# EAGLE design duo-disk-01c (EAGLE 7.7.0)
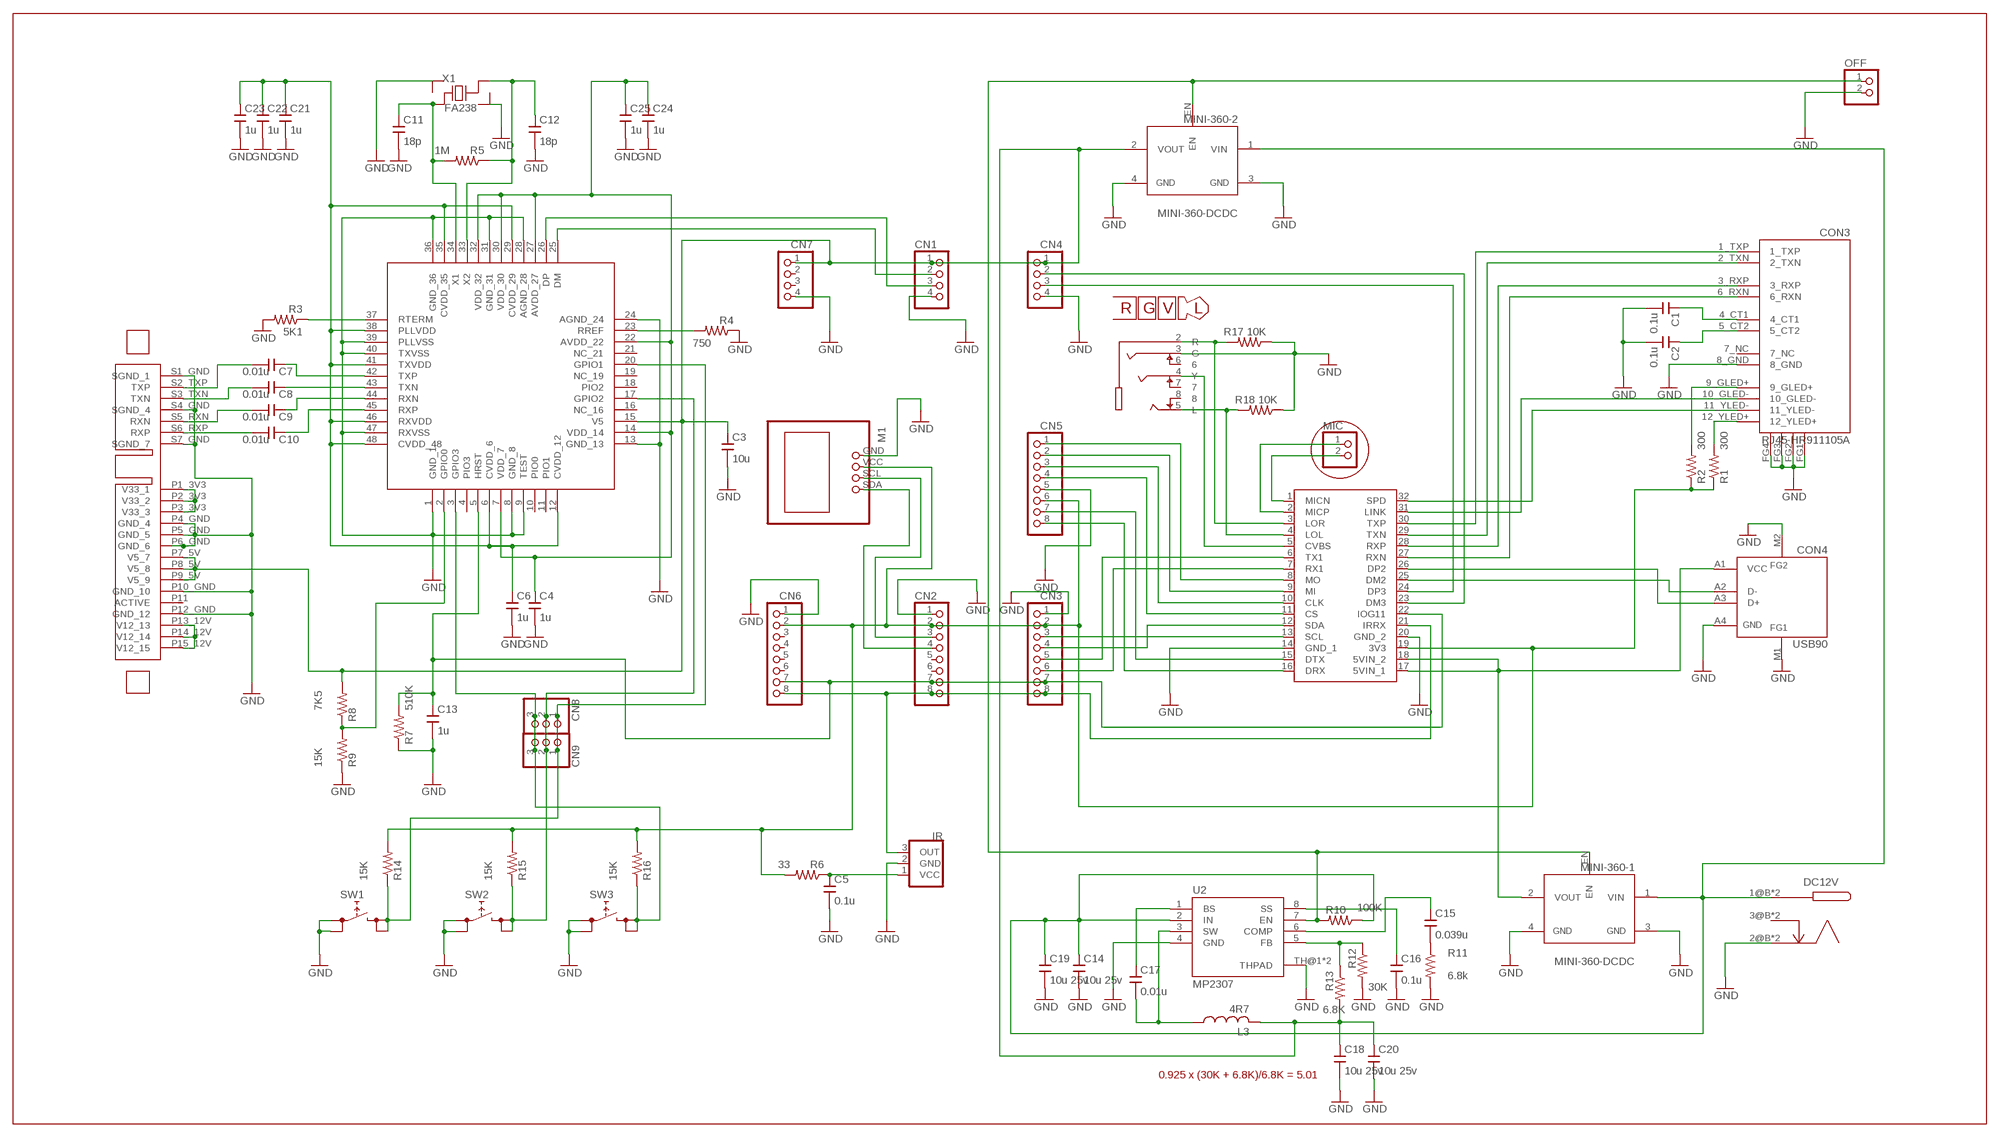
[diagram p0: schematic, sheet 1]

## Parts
C1  0.1u  C/SMDC2012  [C2012]
C2  0.1u  C/SMDC2012  [C2012]
C3  10u  C/SMDC2012  [C2012]
C4  1u  C/SMDC2012  [C2012]
C5  0.1u  C/SMDC2012  [C2012]
C6  1u  C/SMDC2012  [C2012]
C7  0.01u  C/SMDC2012  [C2012]
C8  0.01u  C/SMDC2012  [C2012]
C9  0.01u  C/SMDC2012  [C2012]
C10  0.01u  C/SMDC2012  [C2012]
C11  18p  C/SMDC2012  [C2012]
C12  18p  C/SMDC2012  [C2012]
C13  1u  C/SMDC2012  [C2012]
C14  10u 25v  C/SMDC3216  [C3216]
C15  0.039u  C/SMDC2012  [C2012]
C16  0.1u  C/SMDC2012  [C2012]
C17  0.01u  C/SMDC2012  [C2012]
C18  10u 25v  C/SMDC3216  [C3216]
C19  10u 25v  C/SMDC3216  [C3216]
C20  10u 25v  C/SMDC3216  [C3216]
C21  1u  C/SMDC2012  [C2012]
C22  1u  C/SMDC2012  [C2012]
C23  1u  C/SMDC2012  [C2012]
C24  1u  C/SMDC2012  [C2012]
C25  1u  C/SMDC2012  [C2012]
CN1  CONN4N  [PINHDR1X4]
CN2  PINHDR8  [PINHDR1X8]
CN3  PINHDR8  [PINHDR1X8]
CN4  CONN4N  [PINHDR1X4]
CN5  PINHDR8  [PINHDR1X8]
CN6  PINHDR8  [PINHDR1X8]
CN7  CONN4N  [PINHDR1X4]
CN8  PINHDR3S  [PINHDRS3]
CN9  PINHDR3P  [PADS3]
CON1  SATA-22-07  [SATA-22PIN-A07]
CON2  PJ393  [PJ393]
CON3  RJ45-HR911105A  [RJ45-HR911105A]
CON4  USB90  [USB-AF90]
DC12V  DC-JACK7  [DC-JACK7]
IR  TL1338  [TL1338]
L3  4R7  L/SMD  [L10040]
M1  OLED12864  [OLED12864]
M2  NANOPI-DUO  [NANOPI-DUO]
MIC  PINHDR2  [PINHDR2]
MINI-360-1  MINI-360-DCDC  [MINI-360-DCDC]
MINI-360-2  MINI-360-DCDC  [MINI-360-DCDC]
OFF  PINHDR2  [PINHDR2]
R1  300  R/SMDR2012  [R2012]
R2  300  R/SMDR2012  [R2012]
R3  5K1  R/SMDR2012  [R2012]
R4  750  R/SMDR2012  [R2012]
R5  1M  R/SMDR2012  [R2012]
R6  33  R/SMDR2012  [R2012]
R7  510K  R/SMDR2012  [R2012]
R8  7K5  R/SMDR2012  [R2012]
R9  15K  R/SMDR2012  [R2012]
R10  100K  R/SMDR2012  [R2012]
R11  6.8k  R/SMDR2012  [R2012]
R12  30K  R/SMDR2012  [R2012]
R13  6.8K  R/SMDR2012  [R2012]
R14  15K  R/SMDR2012  [R2012]
R15  15K  R/SMDR2012  [R2012]
R16  15K  R/SMDR2012  [R2012]
R17  10K  R/SMDR2012  [R2012]
R18  10K  R/SMDR2012  [R2012]
SW1  TACTSWSMD+  [TACTSW/SMD+]
SW2  TACTSWSMD+  [TACTSW/SMD+]
SW3  TACTSWSMD+  [TACTSW/SMD+]
U1  GL830  [TQFP48]
U2  MP2307  [SOP8PAD]
X1  FA238  [FA238]

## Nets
CLK: CN5.3 M2.10(CLK)
CS: CN5.4 M2.11(CS)
DM2: CON4.A2(D-) M2.25(DM2)
DM3: CN4.2 M2.23(DM3)
DP2: CON4.A3(D+) M2.26(DP2)
DP3: CN4.3 M2.24(DP3)
DRX: CN5.8 M2.16(DRX)
DTX: CN5.7 M2.15(DTX)
G11: C13.1 CN2.7 CN3.7 CN6.7 M2.22(IOG11) R7.2 U1.5(HRST)
GND: C1.2 C2.2 C3.2 C4.2 C5.2 C6.2 C11.2 C12.2 C13.2 C14.2 C16.2 C18.2 C19.2 C20.2 C21.2 C22.2 C23.2 C24.2 C25.2 CN1.4 CN2.1 CN3.1 CN4.4 CN5.5 CN6.1 CN7.4 CON1.P4_GND(GND_4) CON1.P5_GND(GND_5) CON1.P6_GND(GND_6) CON1.P10_GND(GND_10) CON1.P12_GND(GND_12) CON1.S1_GND(SGND_1) CON1.S4_GND(SGND_4) CON1.S7_GND(SGND_7) CON2.3(G) CON3.8_GND CON3.FG1(GND) CON3.FG2(GND) CON3.FG3(GND) CON3.FG4(GND) CON4.A4(GND) CON4.M1(GND) CON4.M2(GND) DC12V.2@B(GND) DC12V.2@T(GND) IR.2(GND) M1.GND M2.14(GND_1) M2.20(GND_2) MINI-360-1.3(GND) MINI-360-1.4(GND) MINI-360-2.3(GND) MINI-360-2.4(GND) OFF.2 R3.2 R4.1 R7.1 R9.1 R11.2 R12.2 R17.1 R18.1 SW1.1 SW1.2 SW2.1 SW2.2 SW3.1 SW3.2 U1.1(GND_1) U1.8(GND_8) U1.9(TEST) U1.13(GND_13) U1.24(AGND_24) U1.28(AGND_28) U1.31(GND_31) U1.36(GND_36) U1.39(PLLVSS) U1.40(TXVSS) U1.47(RXVSS) U2.4(GND) U2.TH@1(THPAD) U2.TH@2(THPAD) X1.2 X1.4
GPIO0: R8.1 R9.2 U1.2(GPIO0)
GPIO1: CN8.1 CN9.1 R14.1 SW1.3 SW1.4 U1.20(GPIO1)
GPIO2: CN8.2 CN9.2 R15.1 SW2.3 SW2.4 U1.17(GPIO2)
GPIO3: CN8.3 CN9.3 R16.1 SW3.3 SW3.4 U1.3(GPIO3)
IRRX: CN2.8 CN3.8 CN6.8 IR.3(OUT) M2.21(IRRX)
LINK: CON3.10_GLED- M2.31(LINK)
M3V3: CN2.2 CN3.2 CN5.6 CN6.2 M1.VCC M2.19(3V3) R1.1 R2.1 R6.2 R14.2 R15.2 R16.2
M5V: C3.1 C18.1 C20.1 CN1.1 CN4.1 CN7.1 CON1.P7_5V(V5_7) CON1.P8_5V(V5_8) CON1.P9_5V(V5_9) L3.2 L3.2B MINI-360-2.2(VOUT) R8.2 R13.2 U1.15(V5)
MI: CN5.2 M2.9(MI)
MO: CN5.1 M2.8(MO)
N$4: CN1.2 U1.25(DM)
N$7: CN1.3 U1.26(DP)
N$8: CON2.5(L) M2.4(LOL) R18.2
N$9: CON2.4(Y) M2.5(CVBS)
N$10: C17.2 L3.1 L3.1B U2.3(SW)
N$12: CON2.2(R) M2.3(LOR) R17.2
N$13: MINI-360-1.EN MINI-360-2.EN OFF.1 R10.2 U2.7(EN)
N$14: C16.1 U2.8(SS)
N$15: C15.2 R11.1
N$16: C15.1 U2.6(COMP)
N$17: R12.1 R13.1 U2.5(FB)
N$27: M2.2(MICP) MIC.1
N$28: M2.1(MICN) MIC.2
N$30: C7.1 U1.42(TXP)
N$33: C1.1 CON3.4_CT1
N$34: C2.1 CON3.5_CT2
N$36: CON3.9_GLED+ R2.2
N$37: CON3.12_YLED+ R1.2
N$38: CON1.P1_3V3(V33_1) CON1.P2_3V3(V33_2) CON1.P3_3V3(V33_3)
N$39: C17.1 U2.1(BS)
N$41: CON1.P13_12V(V12_13) CON1.P14_12V(V12_14) CON1.P15_12V(V12_15)
N$42: R3.1 U1.37(RTERM)
N$43: R4.2 U1.23(RREF)
N$46: C8.1 U1.43(TXN)
N$47: C7.2 CON1.S2_TXP(TXP)
N$48: C8.2 CON1.S3_TXN(TXN)
N$49: C9.2 CON1.S5_RXN(RXN)
N$50: C10.2 CON1.S6_RXP(RXP)
N$51: C9.1 U1.44(RXN)
N$52: C10.1 U1.45(RXP)
N$53: C11.1 R5.2 U1.34(X1) X1.1
N$54: C12.1 R5.1 U1.33(X2) X1.3
N$61: C5.1 IR.1(VCC) R6.1
OSCL: CN2.3 M1.SCL
OSDA: CN2.4 M1.SDA
RX1: CN3.6 M2.7(RX1)
RXN: CON3.6_RXN M2.27(RXN)
RXP: CON3.3_RXP M2.28(RXP)
S1V8: C6.1 C21.1 C22.1 C23.1 U1.6(CVDD_6) U1.12(CVDD_12) U1.29(CVDD_29) U1.35(CVDD_35) U1.38(PLLVDD) U1.41(TXVDD) U1.46(RXVDD) U1.48(CVDD_48)
S3V3: C4.1 C24.1 C25.1 U1.7(VDD_7) U1.14(VDD_14) U1.22(AVDD_22) U1.27(AVDD_27) U1.30(VDD_30) U1.32(VDD_32)
SCL: CN3.3 M2.13(SCL)
SDA: CN3.4 M2.12(SDA)
SPD: CON3.11_YLED- M2.32(SPD)
TX1: CN3.5 M2.6(TX1)
TXN: CON3.2_TXN M2.29(TXN)
TXP: CON3.1_TXP M2.30(TXP)
VIN: C14.1 C19.1 DC12V.1@B(VIN) DC12V.1@T(VIN) MINI-360-1.1(VIN) MINI-360-2.1(VIN) R10.1 U2.2(IN)
VOUT: CON4.A1(VCC) M2.17(5VIN_1) M2.18(5VIN_2) MINI-360-1.2(VOUT)
Unconnected: CN2.5 CN2.6 CN6.3 CN6.4 CN6.5 CN6.6 CN7.2 CN7.3 CON1.P11(ACTIVE) CON2.6 CON2.7 CON2.8 CON3.7_NC DC12V.3@B(SENSE) DC12V.3@T(SENSE) U1.4(PIO3) U1.10(PIO0) U1.11(PIO1) U1.16(NC_16) U1.18(PIO2) U1.19(NC_19) U1.21(NC_21)

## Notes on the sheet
- 0.925 x (30K + 6.8K)/6.8K = 5.01

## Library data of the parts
C1-C25 = SRT162-020:C/SMD
CN1 CN4 CN7 = SRT162-020:CONN4: connector 4
CN2 CN3 CN5 CN6 = SRT162-020:PINHDR8
CN8 CN9 = SRT162-020:PINHDR3
CON1 = SRT162-020:SATA-22
CON2 = SRT162-020:PJ393
CON3 = SRT162-020:RJ45-HR911105A
CON4 = SRT162-020:USB
DC12V = SRT162-020:DC-JACK
IR = SRT162-020:TL1338
L3 = SRT162-020:L/SMD: VLF4012AT
M1 = SRT162-020:OLED12864
M2 = SRT162-020:NANOPI-DUO
MIC OFF = SRT162-020:PINHDR2
MINI-360-1 MINI-360-2 = SRT162-020:MINI-360-DCDC
R1-R18 = SRT162-020:R/SMD
SW1-SW3 = SRT162-020:TACTSW: 4pin tactsw (1,2 - 3,4)
U1 = SRT162-020:GL830
U2 = SRT162-020:MP2307
X1 = SRT162-020:FA238

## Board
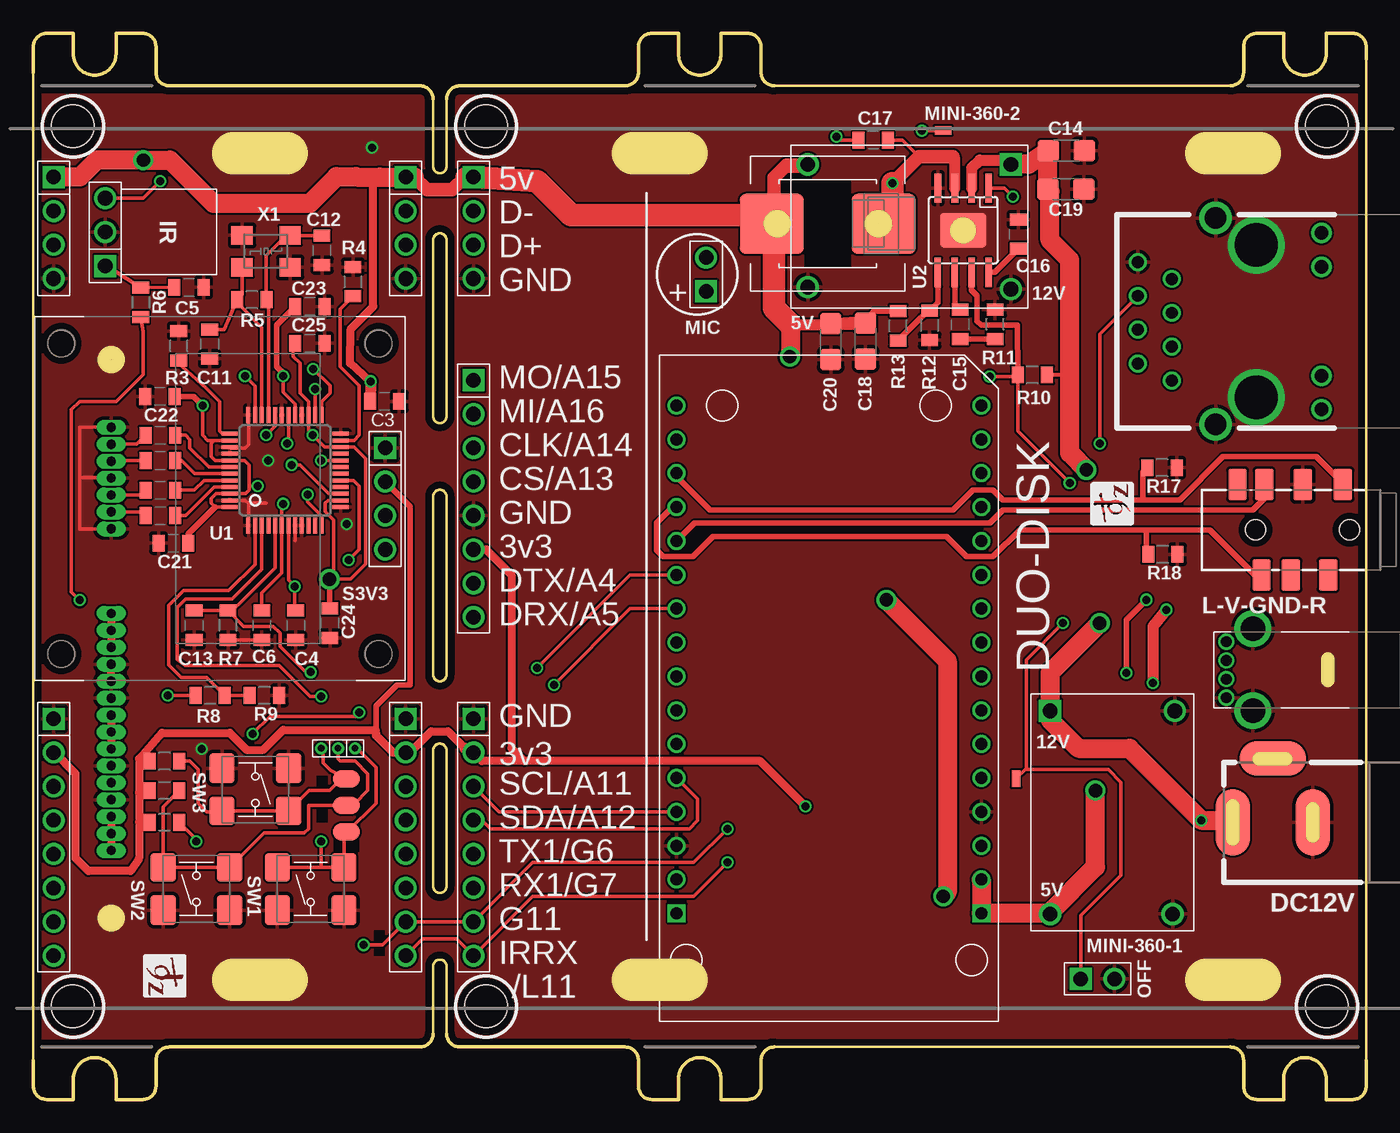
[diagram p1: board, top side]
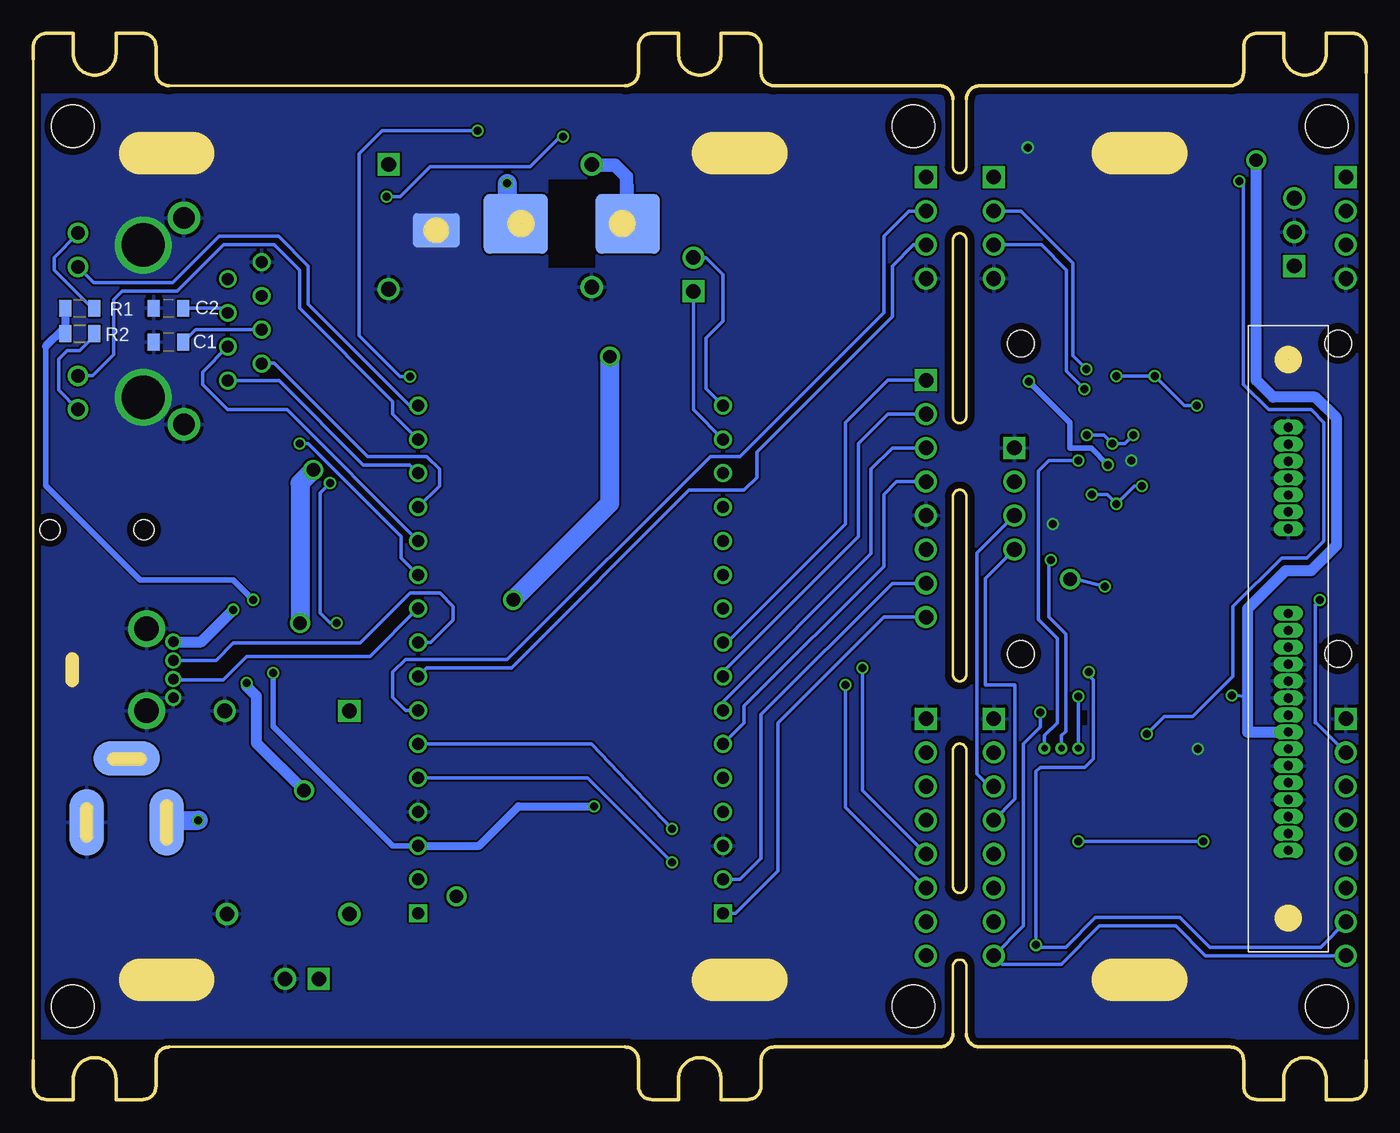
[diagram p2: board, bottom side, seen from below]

Size 100 x 80 mm. Coordinates in mm from the lower left corner, seen from the top.
Outline: 106 segments
Copper layers (1*16): Top 0.035mm / dielectric 1.6mm / Bottom 0.035mm
Design rules "Elecrow_2-layer_PCB_eagle_rule *": minimum track width 6mil, minimum drill 12mil, track to track 6mil, track to pad 6mil, pad to pad 6mil, via to via 8mil, smd to smd 0mil, copper to edge 20mil, drill to drill 10mil, minimum pad ring 8mil, minimum via ring 6mil, stop-mask expansion 0mil, vias tented up to drill 100mil, thermal gap 10mil
Holes 3.2 mm at 2.97,73.02 97.05,73.02 97.05,6.98 2.97,6.98 33.97,73.02 33.97,6.98
tRestrict: area 22.5,18.6 to 24.4,19.4; area 21.3,20.8 to 22.1,22.7; area 25.6,10.8 to 26.4,12.7; area 21.3,22.4 to 22.1,24.3; area -3,75.5 to 104,81; area -4,-1 to 103,4.5
bRestrict: area 21,28.1 to 23.8,29.2; area -3,75.5 to 104,81; area -4,-1 to 103,4.5
Milling: 6 lines

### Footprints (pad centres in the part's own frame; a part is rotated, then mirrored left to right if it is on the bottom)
C2012 = smd 0.9 x 1.25: 1 -1.1,0; 2 1.1,0
C3216 = smd 1.6 x 1.6: 1 -1.35,0; 2 1.35,0
PINHDR1X4 = drill 1.1 square: 1 -3.81,0 | drill 1.1: 2 -1.27,0; 3 1.27,0; 4 3.81,0
PINHDR1X8 = drill 1.1 square: 1 -8.89,0 | drill 1.1: 2 -6.35,0; 3 -3.81,0; 4 -1.27,0; 5 1.27,0; 6 3.81,0; 7 6.35,0; 8 8.89,0
PINHDRS3 = drill 0.5: 1 0,0; 2 1.27,0; 3 2.54,0
PADS3 = smd 1.3 x 2: 1 -2,0; 2 0,0; 3 2,0
SATA-22PIN-A07 = drill 0.7 pad 1.081 long: P1_3V3 0,0; P2_3V3 -1.27,0; P3_3V3 -2.54,0; P4_GND -3.81,0; P5_GND -5.08,0; P6_GND -6.35,0; P7_5V -7.62,0; P8_5V -8.89,0; P9_5V -10.16,0; P10_GND -11.43,0; P11 -12.7,0; P12_GND -13.97,0; P13_12V -15.24,0; P14_12V -16.51,0; P15_12V -17.78,0; S1_GND 13.97,0; S2_TXP 12.7,0; S3_TXN 11.43,0; S4_GND 10.16,0; S5_RXN 8.89,0; S6_RXP 7.62,0; S7_GND 6.35,0
PJ393 = smd 2.4 x 1.4: 2 -3.4,-2.8; 3 -3.4,-5.8; 4 -3.4,-8.7; 5 3.4,-8.9; 6 3.4,-3.9; 7 3.4,-6.7; 8 -3.4,-10.7 | hole 1.5: 0,-2.3; 0,-9.35
RJ45-HR911105A = drill 0.89: 1_TXP 4.45,-6.35; 2_TXN 3.18,-8.89; 3_RXP 1.91,-6.35; 4_CT1 0.64,-8.89; 5_CT2 -0.63,-6.35; 6_RXN -1.9,-8.89; 7_NC -3.17,-6.35; 8_GND -4.44,-8.89 | drill 1.02 pad 1.528: 9_GLED+ 6.625,4.9; 10_GLED- 4.085,4.9; 11_YLED- -4.085,4.9; 12_YLED+ -6.625,4.9 | drill 1.63: FG1 7.745,-3.05; FG2 -7.745,-3.05 | drill 3.25 pad 3.75: FG3 5.715,0; FG4 -5.715,0
USB-AF90 = drill 0.8 pad 1.156: A1 2,-2.1; A2 2,-0.7; A3 2,0.7; A4 2,2.1 | drill 1.84 pad 2.348: M1 0,3.08; M2 0,-3.08
DC-JACK7 = smd 2.6 x 5 bottom: 1@B 4,0; 2@B -2,0 | smd 2.6 x 5: 1@T 4,0; 2@T -2,0 | smd 5 x 2.6 bottom: 3@B 1,-4.8 | smd 5 x 2.6: 3@T 1,-4.8
TL1338 = drill 1.1 square: 1 2.54,0 | drill 1.1: 2 0,0; 3 -2.54,0
L10040 = smd 4.5 x 4.8: 1 0,4.2; 2 0,-4.2 | smd 4.5 x 4.8 bottom: 1B 0,4.2; 2B 0,-4.2
OLED12864 = drill 1.1 square: GND -3.81,0 | drill 1.1: SCL 1.27,0; SDA 3.81,0; VCC -1.27,0 | hole 2: -11.65,-0.5; 11.65,-0.5; -11.65,-24.3; 11.65,-24.3
NANOPI-DUO = drill 0.9: 1 -10.16,10.16; 2 -10.16,7.62; 3 -10.16,5.08; 4 -10.16,2.54; 5 -10.16,0; 6 -10.16,-2.54; 7 -10.16,-5.08; 8 -10.16,-7.62; 9 -10.16,-10.16; 10 -10.16,-12.7; 11 -10.16,-15.24; 12 -10.16,-17.78; 13 -10.16,-20.32; 14 -10.16,-22.86; 15 -10.16,-25.4; 18 12.7,-25.4; 19 12.7,-22.86; 20 12.7,-20.32; 21 12.7,-17.78; 22 12.7,-15.24; 23 12.7,-12.7; 24 12.7,-10.16; 25 12.7,-7.62; 26 12.7,-5.08; 27 12.7,-2.54; 28 12.7,0; 29 12.7,2.54; 30 12.7,5.08; 31 12.7,7.62; 32 12.7,10.16 | drill 0.9 square: 16 -10.16,-27.94; 17 12.7,-27.94
PINHDR2 = drill 1.1 square: 1 -1.27,0 | drill 1.1: 2 1.27,0
MINI-360-DCDC = drill 1.1 pad 1.676 square: 1 -7.62,-5.08 | drill 1.1 pad 1.676: 2 7.62,-5.08; 3 7.62,4.128; 4 -7.62,4.286 | smd 1.27 x 0.66: EN -2.54,-7.62
R2012 = smd 0.9 x 1.25: 1 -1.1,0; 2 1.1,0
TACTSW/SMD+ = smd 2.25 x 1.9: 1 -1.6,2.5; 2 -1.6,-2.5 | smd 2.15 x 1.9: 3 1.6,2.5; 4 1.6,-2.5
TQFP48 = smd 1.2 x 0.3: 1 -4.15,2.75; 2 -4.15,2.25; 3 -4.15,1.75; 4 -4.15,1.25; 5 -4.15,0.75; 6 -4.15,0.25; 7 -4.15,-0.25; 8 -4.15,-0.75; 9 -4.15,-1.25; 10 -4.15,-1.75; 11 -4.15,-2.25; 12 -4.15,-2.75; 25 4.15,-2.75; 26 4.15,-2.25; 27 4.15,-1.75; 28 4.15,-1.25; 29 4.15,-0.75; 30 4.15,-0.25; 31 4.15,0.25; 32 4.15,0.75; 33 4.15,1.25; 34 4.15,1.75; 35 4.15,2.25; 36 4.15,2.75 | smd 0.3 x 1.2: 13 -2.75,-4.15; 14 -2.25,-4.15; 15 -1.75,-4.15; 16 -1.25,-4.15; 17 -0.75,-4.15; 18 -0.25,-4.15; 19 0.25,-4.15; 20 0.75,-4.15; 21 1.25,-4.15; 22 1.75,-4.15; 23 2.25,-4.15; 24 2.75,-4.15; 37 2.75,4.15; 38 2.25,4.15; 39 1.75,4.15; 40 1.25,4.15; 41 0.75,4.15; 42 0.25,4.15; 43 -0.25,4.15; 44 -0.75,4.15; 45 -1.25,4.15; 46 -1.75,4.15; 47 -2.25,4.15; 48 -2.75,4.15
SOP8PAD = smd 0.5 x 2.2: 1 -1.905,-3.154; 2 -0.645,-3.154; 3 0.625,-3.154; 4 1.895,-3.154; 5 1.905,3.154; 6 0.635,3.154; 7 -0.635,3.154; 8 -1.905,3.154 | smd 3.454 x 2.565: TH@1 0,0 | smd 3.454 x 2.565 bottom: TH@2 0,0
FA238 = smd 1.6 x 1.4: 1 -1.8,-1.2; 2 1.8,-1.2; 3 1.8,1.2; 4 -1.8,1.2

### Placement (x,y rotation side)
C1  89.85,56.83 180 bottom
C2  89.85,59.37 180 bottom
C3  26.35,52.39 0 top
C4  19.68,35.58 270 top
C5  11.68,60.94 0 top
C6  17.14,35.58 270 top
C7  9.53,49.85 180 top
C8  9.53,47.94 180 top
C9  9.53,45.72 180 top
C10  9.53,43.81 180 top
C11  13.23,56.69 270 top
C12  21.66,63.72 270 top
C13  12.06,35.58 270 top
C14  77.51,71.2 0 top
C15  69.54,58.16 270 top
C16  73.91,64.94 90 top
C17  63.01,71.98 0 top
C18  62.45,56.91 270 top
C19  77.47,68.29 0 top
C20  59.83,56.85 270 top
C21  10.5,41.75 180 top
C22  9.5,52.75 180 top
C23  20.75,59.5 0 top
C24  22.25,35.75 270 top
C25  20.75,56.75 0 top
CN1  27.94,65.41 270 top
CN2  27.94,19.68 270 top
CN3  33.02,19.68 270 top
CN4  33.02,65.41 270 top
CN5  33.02,45.09 270 top
CN6  1.52,19.68 270 top
CN7  1.52,65.41 270 top
CN8  24.13,26.35 180 top
CN9  23.5,22.07 90 top
CON1  5.84,36.47 90 bottom
CON2  101.05,42.75 270 top
CON3  91.76,58.4 270 top
CON4  91.5,32.25 180 top
DC12V  93.98,20.8 180 top
IR  5.4,65.09 270 top
L3  59.6,65.72 270 top
M1  26.4,45.09 270 top
M2  58.42,41.91 0 top
MIC  50.48,61.91 90 top
MINI-360-1  81.36,21.54 270 top
MINI-360-2  65.72,65.09 180 top
OFF  79.85,9.05 0 top
R1  96.52,59.37 0 bottom
R2  96.52,57.47 0 bottom
R3  10.91,56.56 90 top
R4  23.98,61.37 270 top
R5  16.39,60.02 180 top
R6  8.06,59.8 270 top
R7  14.61,35.58 90 top
R8  13.27,30.32 180 top
R9  17.35,30.32 180 top
R10  74.95,54.38 180 top
R11  72.16,58.17 90 top
R12  67.25,58.08 270 top
R13  64.88,58.06 90 top
R14  9.84,20.8 180 top
R15  9.84,23.18 180 top
R16  9.84,25.4 180 top
R17  84.68,47.41 180 top
R18  84.74,40.91 180 top
SW1  20.81,15.8 90 top
SW2  12.23,15.8 90 top
SW3  16.66,23.25 270 top
U1  18.89,47.21 90 top
U2  69.76,65.22 180 top
X1  17.46,63.64 0 top

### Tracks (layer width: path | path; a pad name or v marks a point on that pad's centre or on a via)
CLK
  Bottom 0.254: M2.10 48.26,29.84 37.15,40.96 37.15,47.31 35.56,48.9 CN5.3
CS
  Bottom 0.254: CN5.4 35.24,46.35 36.2,45.4 36.2,40.01 46.67,29.53 46.67,28.26 M2.11
DM2
  Bottom 0.254: M2.25 70.21,34.29 68.5,36 68.5,37 69.5,38 71.75,38 75.5,34.25 85,34.25 86.3,32.95 CON4.A2
DM3
  Bottom 0.254: M2.23 72.07,29.21 73.03,30.16 73.03,32.07 72.07,33.02 64.45,33.02 49.21,48.26 46.99,48.26 36.2,59.05 36.2,64.77 34.29,66.67 CN4.2
DP2
  Bottom 0.254: CON4.A3 89.45,31.5 85.75,31.5 84,33.25 74.75,33.25 71.17,36.83 M2.26
DP3
  Bottom 0.254: CN4.3 33.97,64.14 35.56,62.55 35.56,58.74 45.72,48.58 45.72,46.67 46.67,45.72 50.8,45.72 64.14,32.38 70.48,32.38 M2.24
DRX
  Bottom 0.254: M2.16 47.31,13.97 44.13,17.14 44.13,28.26 36.2,36.2 CN5.8
DTX
  Bottom 0.254: M2.15 46.99,16.51 45.4,18.1 45.4,28.89 35.56,38.73 CN5.7
G11  (via drill 0.6)
  Top 0.254: v52.07,20.32 49.53,17.78 37.47,17.78 CN3.7 CN2.7 26.19,11.59 v24.77,11.59 | U1.5 18.14,39.88 16.5,38.25 15.75,37.5 14.93,36.68 R7.2 | R7.2 C13.1 | v20.8,32.06 20.44,32.06 18.5,34 18.5,35 18,35.5 15.79,35.5 R7.2
  Bottom 0.254: M2.22 58.1,26.67 v52.07,20.32 | CN6.7 3.42,11.43 11.75,11.43 13.97,13.65 20.32,13.65 22.54,11.43 24.61,11.43 v24.77,11.59 24.77,24.61 24.45,24.92 21.11,24.92 20.48,25.56 20.48,31.48 20.75,31.75 20.74,32 v20.8,32.06
GND  (via drill 0.6)
  Top 0.254: U1.39 14.8,48.9 15.88,48.9 16.14,49.16 U1.36 | U1.40 15.44,48.46 | U1.1 16.14,44.71 | 16.14,44.71 16.19,44.77 17.46,44.77 | U1.47 15.89,44.96 16.14,44.71 | CON1.S1_GND 3.49,50.44 3.49,46.67 | 3.49,46.67 5.84,46.67 CON1.S4_GND | CON1.S7_GND 3.49,42.82 3.49,46.67 | 5.84,22.54 CON1.P12_GND | U1.8 19.64,41.96 | R7.1 C6.2
  Top 0.61: CON1.P5_GND CON1.P4_GND
  other vias: 23.5,43.18 17.62,47.94 12.63,26.3 25.4,71.44
  pour Bottom: -4.45,82.23 -4.45,-4.76 106.05,-4.76 106.05,82.23
  pour Top: -6.03,83.5 -6.03,-2.54 103.5,-2.54 103.5,84.14 -5.71,84.14
GPIO0
  Top 0.254: U1.2 16.64,40.15 14.67,38.19 11.27,38.19 10.16,37.08 10.16,32.61 11.09,31.68 13.01,31.68 R8.1 R9.2
GPIO1  (via drill 0.6)
  Top 0.254: U1.20 21.61,47.96 v21.59,47.94 | CN8.1 24.13,26.51 25.72,24.92 25.72,22.23 23.56,20.07 CN9.1 23.31,19.88 SW1.4 21.59,17.41 | SW1.3 21.59,17.41 | R14.1 12.22,19.52 v12.22,19.37 | v21.59,19.37 21.59,17.41
  Bottom 0.254: v21.59,47.94 23.81,47.94 24.61,47.15 24.61,36.04 23.18,34.61 23.18,28.26 24.13,27.3 CN8.1 | 12.38,19.21 v12.22,19.37 v21.59,19.37
GPIO2  (via drill 0.6)
  Top 0.254: U1.17 24.02,46.46 24.45,46.04 24.45,41.27 v23.65,40.48 | CN8.2 22.86,25.56 23.02,25.4 24.13,25.4 25.08,24.45 25.08,23.18 24.13,22.23 23.65,22.23 CN9.2 | 23.65,22.07 CN9.2 | R15.1 9.73,21.97 SW2.3 SW2.4 17.33,20 20.32,20 20.64,20.32 20.64,22.07 CN9.2
  Bottom 0.254: v23.65,40.48 23.81,40.32 23.81,36.2 22.54,34.92 22.54,27.62 22.86,27.3 CN8.2
GPIO3  (via drill 0.6)
  Top 0.254: U1.3 17.14,39.77 14.92,37.55 11.43,37.55 10.79,36.92 10.79,33.02 11.41,32.56 18.44,32.56 20.75,30.25 21.57,30.25 v21.59,30.23 | CN8.3 21.75,26.19 21.75,25.24 22.29,24.7 CN9.3 23.11,24.07 22.23,23.18 20.69,23.18 SW3.3 SW3.4 14.1,21.59 13.02,21.59 12.38,22.23 12.38,24.77 11.75,25.4 R16.1
  Bottom 0.254: v21.59,30.23 CN8.3
IRRX  (via drill 0.6)
  Top 0.254: v9.53,68.9 8.26,67.63 IR.3 | v52.07,17.78 49.53,15.24 37.47,15.24 CN3.8 31.75,12.06 29.21,12.06 CN2.8 | v24.45,29.03 24.17,28.75 17.75,28.75 16.46,27.46 v16.46,27.44
  Bottom 0.254: v24.45,29.03 24.45,27.96 25.72,26.69 25.72,13.02 CN2.8 27.3,10.16 22.86,10.16 20,13.02 14.29,13.02 12.06,10.79 CN6.8 | v9.53,68.9 9.21,68.9 9.21,53.66 7.3,51.75 4.13,51.75 3.17,50.8 3.17,41.91 4.45,40.64 6.35,40.64 10,36.99 10,31.75 13,28.75 15.15,28.75 v16.46,27.44 | M2.21 58.42,24.13 v52.07,17.78
LINK
  Bottom 0.254: M2.31 73.03,51.44 73.03,52.39 80.01,59.37 80.01,62.23 81.92,64.14 85.72,64.14 89.22,60.64 93.34,60.64 93.98,60.01 93.98,55.88 95.55,54.31 CON3.10_GLED-
M3V3  (via drill 0.6)
  Top 0.254: 1.59,26.04 CN6.2 | R6.2 8.26,57.64 8.26,54.41 6.24,52.39 3.49,52.39 2.86,51.75 2.86,38.1 v3.49,37.47
  Top 0.406: M1.VCC 28.26,44.5 28.26,31.11 27.3,31.11 25.72,29.53 25.72,27.51 | v82,32 82,36 v83.5,37.5
  Top 0.61: 7.94,25.56 7.94,23.02 | 7.94,23.02 7.94,20.8 | 7.94,20.8 7.94,18.1 7.3,17.14 4.13,17.14 3.17,18.1 3.17,24.45 1.59,26.04 | 25.72,27.3 25.72,27.51 | R16.2 8.1,25.4 7.94,25.56 | R15.2 8.1,23.18 7.94,23.02 | R14.2 7.94,20.8 | 25.72,27.3 26.99,26.04 CN2.2 | 36.83,25.4 54.53,25.4 v57.93,22 | 36.83,25.4 33.66,25.4 CN3.2 | CN5.6 33.97,41.27 35.88,39.37 35.88,26.35 36.83,25.4 | 28.26,26.04 29.84,27.62 31.11,27.62 32.38,26.35 | 7.94,25.56 9.64,27.51 14.74,27.51 16,26.25 17.25,26.25 18.75,27.75 25.66,27.75 25.72,27.3
  Top 0.813: CN2.2 28.26,26.04 | 32.38,26.35 32.7,26.35 CN3.2
  Bottom 0.254: v3.49,37.47 3.81,37.15 3.81,28.26 3.74,28.26 CN6.2 | R2.1 97.79,57.78
  Bottom 0.406: M2.19 73.05,19.05 82,28 v82,32 | v83.5,37.5 85,39 92,39 99.06,46.06 99.06,56.52
  Bottom 0.61: R1.1 R2.1 | 97.79,57.78 99.06,56.52 | M2.19 66.55,19.05 63.6,22 v57.93,22
M5V  (via drill 0.6, 1)
  Top 0.254: U1.15 22.17,45.46 20,47.62 v19.37,47.62 | R8.2 v10.09,30.32 | 55.24,67.31 55.4,67.15 L3.2B
  Top 0.406: R13.2 63.05,59.16 C18.1 62.3,58.15
  Top 0.61: CON1.P7_5V CON1.P8_5V CON1.P9_5V | 23.81,68.9 24.25,69.22 | v25.31,53.89 25.25,53.89 23.75,55.25 23.81,57.81 25.5,59.5 25.5,68.97 26,69.22 | L3.2B 55.4,69.06 55.56,69.22 | 55.56,69.22 55.88,69.22 56.52,69.85 57.78,69.85 MINI-360-2.2 56.52,70.17 55.56,69.22 | 55.56,69.22 55.56,66.36
  Top 0.813: v25.31,53.89 C3.1 | C20.1 62.64,58.45 C18.1 | 62.3,58.15 59.72,58.15 59.67,58.1 56.83,58.1
  Top 1.016: 28.57,69.22 29.53,68.26 31.43,68.26 32.38,69.22 | 55.56,65.56 55.56,66.36 55.56,69.17 56.5,70.1 58.04,70.1 MINI-360-2.2
  Top 1.422: CN7.1 3.49,69.22 4.76,70.48 v8.26,70.48 10.27,70.48 13.5,67.25 20.75,67.25 22.75,69.25 24.21,69.25 24.25,69.22 26,69.22 CN1.1 28.57,69.22 | 32.38,69.22 CN4.1 | v68.26,15.24 68.58,15.56 68.58,32.92 v64,37.5 | v56.75,55.75 56.83,55.83 56.83,58.1
  Top 1.676: CN4.1 37.78,68.9 40.33,66.35 55.56,66.36 | 56.83,58.1 55.56,59.37 55.56,65.56
  Bottom 0.254: v10.09,30.32 9.96,30.32 8.89,30.25
  Bottom 0.406: v25.31,53.89 22.23,50.8 22.23,48.9 20.64,48.9 v19.37,47.62
  Bottom 0.61: L3.2B 54.94,65.72 54.93,65.72 54.93,66.04 55.24,66.36 55.24,68.58 55.56,68.9 55.56,69.17 56.38,69.98 57.92,69.98 MINI-360-2.2
  Bottom 0.813: v8.26,70.48 8.26,53.98 6.99,52.7 3.81,52.7 2.22,51.12 2.22,41.59 4.13,39.69 6.03,39.69 8.89,36.83 8.89,30.25 8.89,27.58 CON1.P8_5V
  Bottom 1.016: 55.25,65.87 L3.2B | 58.06,70.1 56.35,70.1 55.5,69.25 55.5,65.81 L3.2B | L3.2B 55.4,66.09 55.56,66.25 55.56,65.88 L3.2B
  Bottom 1.422: v64,37.5 56.75,44.75 v56.75,55.75
MI
  Bottom 0.254: M2.9 48.26,32.07 38.1,42.23 38.1,49.21 35.88,51.44 CN5.2
MO
  Bottom 0.254: M2.8 47.94,34.29 39.05,43.18 39.05,50.8 35.88,53.98 CN5.1
N$4  (via drill 0.6)
  Top 0.254: U1.25 21.64,52.39 22.25,53 22.25,53.56 v21,54.81
  Bottom 0.254: v21,54.81 22,55.81 22,62.75 25.93,66.67 CN1.2
N$7  (via drill 0.6)
  Top 0.254: U1.26 v21.14,53.29
  Bottom 0.254: CN1.3 24.39,64.14 22.5,62.25 22.5,54.66 v21.14,53.29
N$8
  Top 0.406: CON2.5 91.65,39.35 88.25,42.75 83.5,42.75 | M2.4 47.95,44.45 46.75,43.25 46.75,41.25 47.25,40.75 49.5,40.75 51,42.25 68.5,42.25 70,40.75 72,40.75 74,42.75 83.5,42.75 | R18.2 83.5,41.55 83.5,42.75
N$9
  Top 0.254: CON2.4 92.35,45.6
  Top 0.406: 92.35,45.6 92.35,45.1 91.5,44.25 72.75,44.25 71.75,43.25 49.6,43.25 M2.5
N$10  (via drill 0.6)
  Top 0.254: L3.1B 63.82,65.73 63.82,67.63 64.45,68.26 v64.45,68.75 | 66.46,70.75 65.22,71.98 C17.2
  Top 0.406: 64.45,66.36 L3.1B
  Top 0.61: 69.14,70.61 69,70.75
  Top 0.813: 64.45,68.9 v64.45,68.75 | U2.3 69.14,70.61
  Top 1.016: 69,70.75 66.46,70.75 v64.45,68.75
  Top 1.676: 64.45,68.58 v64.45,68.75 64.45,66.36
  Bottom 0.152: 63.86,65.84 L3.1B
  Bottom 1.422: v64.45,68.75 64.45,66.36 L3.1B
N$12
  Top 0.254: CON2.2 98.25,46.25
  Top 0.406: 98.25,46.25 96.25,48.25 89.25,48.25 86,45 83.25,45 | 48.51,46.99 M2.3 48.26,46.74 50.75,44.25 69,44.25 70.5,45.75 72,45.75 72.75,45 83.25,45 | R17.2 83.25,47.08 83.25,45
N$13  (via drill 0.6)
  Top 0.254: 73.73,24.36 MINI-360-1.EN | MINI-360-1.EN 73.85,24.2 | 73.85,54 73.85,50.15 v77.75,46.25 | 73.85,54 R10.2 | MINI-360-2.EN v66.67,72.71 | OFF.1 78.58,13.81 81.6,16.83 81.6,23.81 80.64,24.77 74.42,24.77 MINI-360-1.EN | MINI-360-1.EN 74.5,24.84 74.5,33 v77.25,35.75 | v71.75,54.25 73.6,54.25 73.85,54
  Top 0.406: U2.7 70.4,60.73 70.8,60.33 70.8,58.42 71.12,58.1 73.83,58.1 R10.2
  Bottom 0.254: v66.67,72.71 73.82,72.71 75.56,70.96 75.56,57.31 72.5,54.25 v71.75,54.25 | v77.75,46.25 78.5,45.5 78.5,36.5 77.75,35.75 v77.25,35.75
N$14
  Top 0.406: U2.8 72.14,62.07 C16.1
N$15
  Top 0.406: C15.2 71.89,57.06 R11.1
N$16
  Top 0.406: U2.6 69.13,59.67 C15.1
N$17
  Top 0.406: U2.5 67.86,59.79 R12.1 66.6,58.68 R13.1
N$27
  Bottom 0.254: M2.2 50.48,51.75 MIC.1
N$28
  Bottom 0.254: M2.1 49.53,53.34 49.53,57.15 48.26,58.42 48.26,61.91 49.53,63.18 MIC.2
N$30
  Top 0.254: U1.42 13.18,47.46 11.75,48.9 11.75,49.53 11.43,49.85 C7.1
N$33
  Bottom 0.254: CON3.4_CT1 87.83,57.76 C1.1
N$34
  Bottom 0.254: CON3.5_CT2 85.75,59.37 C2.1
N$36
  Bottom 0.254: 95.57,57.47 R2.2 95.42,57.3 96.52,56.2 97.47,56.2 98.11,55.56 98.11,53.23 CON3.9_GLED+
N$37
  Bottom 0.254: R1.2 95.57,59.37 98.42,62.23 98.42,63.18 96.66,64.95 CON3.12_YLED+
N$38
  Top 0.61: CON1.P1_3V3 CON1.P2_3V3 CON1.P3_3V3
N$39  (via drill 0.6)
  Top 0.254: U2.1 72.87,68.38 v73.5,67.75 | 61.89,72.25 C17.1 60.52,71.98 v60.25,72.25
  Bottom 0.254: v73.5,67.75 72.5,67.75 70.25,70 62.75,70 60.5,72.25 v60.25,72.25
N$41
  Top 0.61: CON1.P13_12V CON1.P14_12V CON1.P15_12V
N$42
  Top 0.254: U1.37 14.18,49.96 13.97,50.16 13.97,52.39 13.02,53.34 10.79,55.34 10.91,55.48 R3.1
N$43
  Top 0.254: U1.23 24.06,49.46 24.45,49.85 24.45,53.55 23,55 23,59.29 R4.2
N$46
  Top 0.254: U1.43 12.1,46.96 11.11,47.94 C8.1
N$47
  Top 0.254: C7.2 7.75,49.17 CON1.S2_TXP
N$48
  Top 0.254: CON1.S3_TXN 5.88,47.94 C8.2
N$49
  Top 0.254: C9.2 8.06,45.36 CON1.S5_RXN
N$50
  Top 0.254: C10.2 8.15,44.09 CON1.S6_RXP
N$51
  Top 0.254: U1.44 12.8,46.46 12.06,45.72 C9.1
N$52
  Top 0.254: U1.45 13.57,45.96 11.43,43.81 C10.1
N$53
  Top 0.254: U1.34 17.14,57.94 15.29,59.78 R5.2 | C11.1 14.32,57.79 R5.2 | R5.2 15.66,60.38 X1.1
N$54
  Top 0.254: U1.33 17.64,59.87 R5.1 17.46,60.3 17.46,63.33 18.73,64.59 19.02,64.59 X1.3 19.29,64.81 C12.1
N$61
  Top 0.254: C5.1 R6.1 5.54,62.55 IR.1
OSCL
  Bottom 0.254: M1.SCL 29.21,41.01 29.21,24.45 28.26,23.5 CN2.3
OSDA
  Bottom 0.254: M1.SDA 28.57,39.1 28.57,31.11 26.35,31.11 26.35,22.54 CN2.4
RX1  (via drill 0.6)
  Top 0.254: M2.7 44.77,36.83 v39.05,31.11
  Bottom 0.254: v39.05,31.11 39.05,21.91 CN3.6
RXN  (via drill 0.6)
  Top 0.254: v80.01,49.21 80.01,57.44 CON3.6_RXN
  Bottom 0.254: M2.27 72.39,40.64 72.39,42.23 79.38,49.21 v80.01,49.21
RXP
  Bottom 0.254: M2.28 80.96,51.75 85.41,51.75 87.31,53.66 87.31,54.59 CON3.3_RXP
S1V8  (via drill 0.6)
  Top 0.254: U1.48 13.64,44.46 13.34,44.77 13.34,45.09 13.71,45.46 U1.46 15.93,45.46 16.19,45.72 16.19,46.04 | 13.58,49.46 13.34,49.21 13.34,48.26 13.63,47.96 U1.41 15.86,47.96 16.19,47.62 16.19,46.04 | U1.38 13.58,49.46 | v18.73,44.7 18.64,44.35 U1.6 18.64,39.5 17.14,38.01 C6.1 | v16.83,46.04 16.19,46.04 | U1.12 21.64,43.77 20.57,44.84 v20.57,45.4 | 13.58,49.46 13.09,49.46 12.7,49.85 v12.7,52.07 | U1.35 16.64,53.53 v15.88,54.29 | U1.29 19.64,52.19 18.73,53.09 v18.73,54.29
  Top 0.406: C21.1 11.6,42.42 13.64,44.46 | C22.1 12.02,52.75 v12.7,52.07 | C23.1 18.25,58.1 18.25,55 18.73,54.52 v18.73,54.29
  Bottom 0.254: v16.83,46.04 17.39,46.04 v18.73,44.7 19.43,45.4 v20.57,45.4 | v18.73,54.29 v15.88,54.29 13.65,52.07 v12.7,52.07
S3V3  (via drill 0.6, 1.02)
  Top 0.254: U1.32 18.14,50.52 v17.46,49.85 | U1.7 19.14,38.98 v19.62,38.51 19.62,36.75 C4.1 | U1.30 19.14,49.3 v19.05,49.21 | U1.14 22.1,44.96 21.91,44.77 21.91,44.13 22.54,43.5 22.54,39.37 v22.23,39.05 | 23.02,39.05 v22.23,39.05 | v22.23,39.05 23.81,39.05 24.92,40.16 24.92,48.1 24.07,48.96 U1.22 21.84,48.96 v20.95,49.85 20.64,50.16 U1.27 20.64,52.36 20,53 20,55.25 19.5,55.75 19.5,56.85 C25.1
  Top 0.406: C24.1 22.23,36.88 v22.23,39.05
  Bottom 0.254: v17.46,49.85 18.1,49.21 v19.05,49.21 19.68,49.85 v20.95,49.85 | v22.23,39.05 21.66,39.01 v19.62,38.51
SCL
  Top 0.254: M2.13 34.92,21.59 CN3.3
SDA
  Top 0.254: M2.12 49.85,22.54 49.85,20.95 49.21,20.32 34.29,20.32 33.66,20.95 CN3.4
SPD
  Bottom 0.254: M2.32 71.75,52.07 79.38,59.69 79.38,62.55 81.6,64.77 86.04,64.77 89.53,61.28 95.45,61.28 CON3.11_YLED-
TX1  (via drill 0.6)
  Top 0.254: M2.6 47.94,39.05 47.62,39.37 44.77,39.37 v37.78,32.38
  Bottom 0.254: v37.78,32.38 37.78,23.18 CN3.5
TXN
  Bottom 0.254: M2.29 69.53,46.04 69.53,47.31 70.48,48.26 74.93,48.26 81.92,55.24 82.84,55.24 CON3.2_TXN
TXP
  Bottom 0.254: M2.30 71.75,47.62 75.25,47.62 81.57,53.95 CON3.1_TXP
VIN  (via drill 0.6, 1)
  Top 0.305: R10.1 77.62,54.38 77.75,54.25
  Top 0.61: 76.28,28.5 MINI-360-1.1 | 76.12,70.91 C14.1 | 73.01,70.5 MINI-360-2.1
  Top 0.813: U2.2 70.41,69.91 71,70.5 73.01,70.5
  Top 1.422: 76.28,28.5 78.42,26.35 82.23,26.35 v87.63,20.95 89.83,20.95 DC12V.1@B | 76.12,70.91 C19.1 76.28,68.14 76.28,64.47 77.75,63 77.75,54.25 77.75,48.5 v79,47.25 | C14.1 74.69,70.17 MINI-360-2.1 | v80,35.75 76.28,32.02 MINI-360-1.1
  Bottom 0.152: 89,20.88 89.92,20.88 DC12V.1@B
  Bottom 1.422: DC12V.1@B 89.83,20.95 v87.63,20.95 | v79,47.25 80,46.25 v80,35.75
VOUT  (via drill 0.6, 1)
  Top 0.61: MINI-360-1.2 76.22,13.97
  Top 0.813: v85,36.75 84,35.5 v84,31.25
  Top 1.422: M2.18 M2.17 76.22,13.97 79.69,17.44 v79.69,23.18
  Bottom 0.61: 84,31 v84,31.25
  Bottom 0.813: CON4.A1 87.4,34.35 v85,36.75 | v79.69,23.18 83.25,26.73 83.25,30.25 84,31

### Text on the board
tPlace: 5v | D- | D+ | GND | + | 12V | 5V | MO/A15 | MI/A16 | CLK/A14 | CS/A13 | GND | 3v3 | DTX/A4 | S3V3 | DRX/A5 | L-V-GND-R | DUO-DISK | GND | 12V | 3v3 | SCL/A11 | SDA/A12 | TX1/G6 | RX1/G7 | 5V | G11 | IRRX | /L11
tDocu: PWRLED-L10 | STATLED-A10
